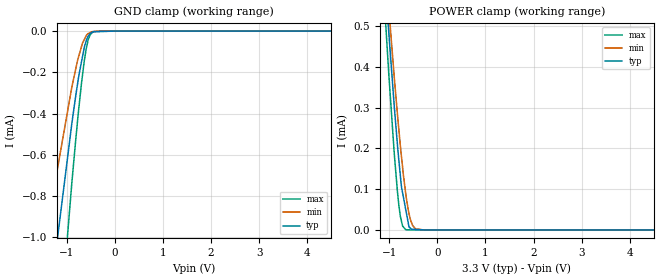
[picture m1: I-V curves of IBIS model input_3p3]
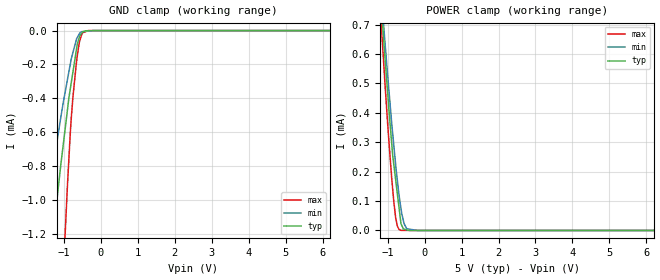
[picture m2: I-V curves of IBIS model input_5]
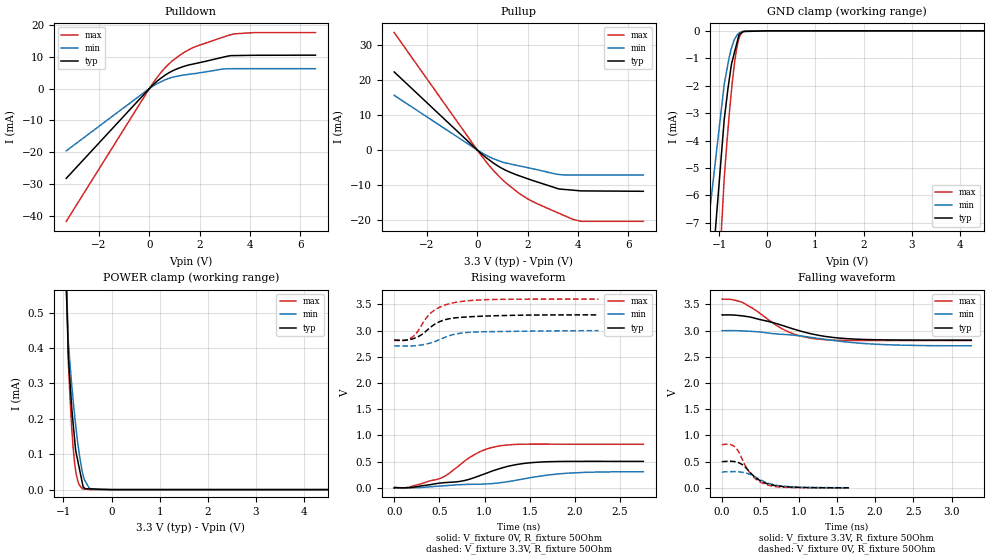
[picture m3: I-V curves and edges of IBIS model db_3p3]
|Texas Instruments Incorporated
| 16-Bit, 2MSPS ADC with P8/P16 Parallel Output, Internal Clock & Internal
| Reference
| Marketing part#   Digital Voltage Range   Package-type   #pins
| ADS8411IBPFBR   2.7V - 5.25V   TQFP   48
| ADS8411IBPFBRG4   2.7V - 5.25V   TQFP   48
| ADS8411IBPFBT   2.7V - 5.25V   TQFP   48
| ADS8411IBPFBTG4   2.7V - 5.25V   TQFP   48
| ADS8411IPFBT   2.7V - 5.25V   TQFP   48
| ADS8411IPFBTG4   2.7V - 5.25V   TQFP   48
[IBIS Ver]   3.2
[File name]   ads8411.ibs
|SIMDE Ver   V3.0 - 201101 - RHL4 - Build 457
[File Rev]   1.0
[Date]   7/21/2011
[Source]
| Texas Instruments Incorporated.
| Analog-eLab Design Center, HPA
| 12500 TI Blvd
| Dallas, TX -75243
| e-mail: elab_scm_ibis@list.ti.com
[Notes]   Revision History:
| Rev 1.0: 7/21/2011
| - Initial version of the model
| - Model generated from simulations in TISPICE
| - Model matched to SPICE simulation
| - C_comp although listed in numerical order of value are
|   obtained from varying PVT conditions. For PVT conditions for
|   each specific value refer the buffer description under
|   respective [Model]. IBIS model user is responsible for using
|   appropriate C_comp to simulate for Signal Integrity.
| - Model names with a trailing _3p3 contains the model for
|   3.3V [3.0V and 3.6V]. Model names with a trailing _5 contains
|   the model for 5.0V [4.5V and 5.5V].
| - Relative part of ADS8412.
|*   EXCEPTION:   *
|*   - Because of the resistor network connected to pad,there will  *
|*   be a leakage current in the Pullup table MAX corner of busy_5*
|*   & POWER CLAMP IV table MAX corners db_5 and db4to11_5 models.*
[Disclaimer]
| This model is designed as an aid for customers of Texas Instruments.
| TI and its licensors and suppliers make no warranties, either expressed
| or implied, with respect to this  model, including the warranties of
| merchantability or fitness for a particular purpose. The model is
| provided solely on an "as is" basis. The entire risk as to its quality
| and performance is with the customer.
[Copyright]
 (C) Copyright 2011 Texas Instruments Incorporated.All rights reserved.
|   ADS8411
[Component]   ADS8411
[Manufacturer]   TI
[Package]   |48 TQFP   -  PFB package
|   typ   min   max
R_pkg   0.07474   0.04062   0.08595
L_pkg   2.62799nH   2.23868nH   3.44226nH
C_pkg   0.45808pF   0.38230pF   0.56945pF
[Pin]  signal_name   model_name   R_pin   L_pin   C_pin
1   REFIN   TERM   0.08206   3.37721nH  0.55796pF
2   REFOUT   TERM   0.07311   2.63474nH  0.48712pF
3   NC   NC   0.06827   2.49388nH  0.46543pF
4   VA+   POWER   0.06574   2.45218nH  0.45840pF
5   AGND   GND   0.06538   2.26018nH  0.41356pF
6   IN+   TERM   0.06584   2.24077nH  0.38230pF
7   IN-   TERM   0.06683   2.25918nH  0.38313pF
8   AGND   GND   0.06727   2.29722nH  0.41664pF
9   VA+   POWER   0.07011   2.54080nH  0.46468pF
10   VA+   POWER   0.07450   2.61853nH  0.47441pF
11   AGND   GND   0.08090   2.78937nH  0.50097pF
12   AGND   GND   0.02781   2.88082nH  0.62037pF
13   VA+   POWER   0.08724   3.49123nH  0.55959pF
14   AGND   GND   0.08150   2.80909nH  0.48998pF
15   AGND   GND   0.08471   2.82596nH  0.47804pF
16   DB15   DB   0.08265   2.78879nH  0.47897pF
17   DB14   DB   0.08081   2.56943nH  0.43166pF
18   DB13   DB   0.08007   2.52568nH  0.39763pF
19   DB12   DB   0.07920   2.50619nH  0.39700pF
20   DB11   DB4to11   0.07811   2.51437nH  0.42861pF
21   DB10   DB4to11   0.07805   2.69832nH  0.47285pF
22   DB9   DB4to11   0.07892   2.71042nH  0.47434pF
23   DB8   DB4to11   0.08131   2.80113nH  0.49547pF
24   VBD+   POWER   0.08699   3.47547nH  0.56533pF
25   BDGND   GND   0.09181   3.57831nH  0.56951pF
26   DB7   DB4to11   0.08145   2.80544nH  0.49887pF
27   DB6   DB4to11   0.07496   2.62998nH  0.47483pF
28   DB5   DB4to11   0.07046   2.54788nH  0.46573pF
29   DB4   DB4to11   0.06751   2.30378nH  0.41738pF
30   DB3   DB   0.06637   2.25187nH  0.38313pF
31   DB2   DB   0.06583   2.23868nH  0.38275pF
32   DB1   DB   0.06587   2.26752nH  0.41559pF
33   DB0   DB   0.06778   2.49130nH  0.46143pF
34   VBD+   POWER   0.07134   2.55123nH  0.46971pF
35   BDGND   GND   0.07672   2.70037nH  0.49534pF
36   BUSY   BUSY   0.08595   3.44226nH  0.56945pF
37   VBD+   POWER   0.08902   3.51744nH  0.56277pF
38   _RESET   INPUT   0.08223   2.81495nH  0.49515pF
39   BYTE   INPUT   0.07913   2.70647nH  0.47619pF
40   _CONVST   INPUT   0.07793   2.68782nH  0.47314pF
41   _RD   INPUT   0.07804   2.50508nH  0.42870pF
42   _CS   INPUT   0.07951   2.50501nH  0.39774pF
43   VA+   POWER   0.08105   2.53403nH  0.39929pF
44   AGND   GND   0.08220   2.58618nH  0.42997pF
45   AGND   GND   0.07817   2.69201nH  0.46931pF
46   VA+   POWER   0.07884   2.69863nH  0.47572pF
47   REFM   TERM   0.04062   2.38885nH  0.53583pF
48   REFM   TERM   0.08222   3.37069nH  0.56325pF
|   Model Selectors
[Model Selector] INPUT
input_3p3  3.3V digital input
input_5   5.0V digital input
[Model Selector] BUSY
busy_3p3   3.3V digital output
busy_5   5.0V digital output
[Model Selector] DB
db_3p3   3.3V 3-state output
db_5   5.0V 3-state output
[Model Selector] DB4to11
db4to11_3p3   3.3V 3-state output
db4to11_5   5.0V 3-state output
[Model Selector] TERM
term_3-3V  3.3V nominal termination
term_5-0V  5.0V nominal termination
[Model] term_3-3V
Model_type Terminator
C_comp   1.0e-20F  1.0e-20F  1.0e-20F
|   typ   min   max
[Voltage Range]   3.3V   3.0V   3.6V
[POWER Clamp Reference]   3.3V   3.0V   3.6V
[GND Clamp Reference]   0V   0V   0V
|Ambient Temperature   25   85   -40
|Junction Temperature
[Temperature Range]   40   100   -40
[Model] term_5-0V
Model_type Terminator
C_comp   1.0e-20F  1.0e-20F  1.0e-20F
|   typ   min   max
[Voltage Range]   5.0V   4.75V   5.25V
[POWER Clamp Reference]   5.0V   4.75V   5.25V
[GND Clamp Reference]   0V   0V   0V
|Ambient Temperature   25   85   -40
|Junction Temperature
[Temperature Range]   40   100   -40
| Models and submodels in the file (10): input_3p3 (Input), input_5 (Input), db_3p3 (3-state), db_5 (3-state), db4to11_3p3 (3-state), db4to11_5 (3-state), busy_3p3 (Output), busy_5 (Output), term_3-3V (Terminator), term_5-0V (Terminator)
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|   input_3p3 Model
[Model]   input_3p3
Model_type   Input
Vinl = 0.8
Vinh = 2.3
|   typ   min   max
|   (nom PVT)   (fast PVT)   (slow PVT)
|C_comp from frequency sweep method (F=1MHz)
|Average
|C_comp   2.437e-12   2.379e-12   2.445e-12
|C_comp from LC tank measurement(L=1nH)
|Average
|Resonant Frequency(Hz)   3.580e+09   3.600e+09   3.550e+09
C_comp   1.978e-12   1.956e-12   2.012e-12
| Where nom  PVT is Nominal Process, 3.3V, 40C
|   Fast PVT is Strong Process,  3.6V, -40C
|   Slow PVT is Weak Process,   3V, 100C
[Model Spec]
Vinh   2.3   2.0   2.6
[Voltage Range]   3.3   3   3.6
|Ambient Temperature   25   85   -40
|Junction Temperature
[Temperature Range]   40   100   -40
[Power Clamp Reference]   3.3   3   3.6
[GND Clamp Reference]   0   0   0
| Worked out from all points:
|   GND clamp passes 1 mA (typ) near -1.19 V on its own axis
|   POWER clamp passes 1 mA (typ) near -1.31 V on its own axis
[GND Clamp]
|   Voltage   I(typ)   I(min)   I(max)
-3.3V     -5.989mA   -4.026mA   -11.09mA
-1.561V   -1.759mA   -1.203mA   -2.732mA
-1.26V    -1.141mA   -754.9uA   -1.788mA
-1.191V   -999.8uA   -663.8uA   -1.581mA
-897.6mV  -451.9uA   -274.2uA   -742.2uA
-752.4mV  -219.8uA   -122.3uA   -378.7uA
-691.2mV  -145.1uA   -72.4uA    -245.9uA
-640.8mV  -84.92uA   -42.96uA   -151.8uA
-597.6mV  -48.27uA   -23.13uA   -86.98uA
-558mV    -25.78uA   -12.14uA   -44.62uA
-471mV    -5.465uA   -2.721uA   -6.698uA
6.6V      0A         0A         0A
[POWER Clamp]
|   Voltage   I(typ)   I(min)   I(max)
-3.3V     4.863mA    4.572mA    5.323mA
-1.159V   738uA      777.9uA    667uA
-1.035V   523.5uA    580.1uA    428.9uA
-1.012V   486uA      545.3uA    384uA
-896.4mV  302.7uA    373.8uA    186.6uA
-802.8mV  172.8uA    247.7uA    62.16uA
-745.8mV  104.9uA    178.4uA    20.9uA
-658.8mV  50.38uA    89.49uA    921.5nA
-590.7mV  7.702uA    39.87uA    227.2nA
-513mV    1.843uA    10.64uA    0A
-285mV    155.8nA    42.15nA    0A
6.6V      0A         0A         0A
|   input_5 Model
[Model]   input_5
Model_type   Input
Vinl = 0.8
Vinh = 4.0
|   typ   min   max
|   (nom PVT)   (fast PVT)   (slow PVT)
|C_comp from frequency sweep method (F=1MHz)
|Average
|C_comp   2.380e-12   2.336e-12   2.422e-12
|C_comp from LC tank measurement(L=1nH)
|Average
|Resonant Frequency(Hz)   3.580e+09   3.600e+09   3.550e+09
C_comp   1.978e-12   1.956e-12   2.012e-12
| Where nom  PVT is Nominal Process, 5V, 40C
|   Fast PVT is Strong Process,  5.25V, -40C
|   Slow PVT is Weak Process,   4.75V, 100C
[Model Spec]
Vinh   4.0   3.75   4.25
[Voltage Range]   5   4.75   5.25
|Ambient Temperature   25   85   -40
|Junction Temperature
[Temperature Range]   40   100   -40
[Power Clamp Reference]   5   4.75   5.25
[GND Clamp Reference]   0   0   0
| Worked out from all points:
|   GND clamp passes 1 mA (typ) near -1.19 V on its own axis
|   POWER clamp passes 1 mA (typ) near -1.31 V on its own axis
[GND Clamp]
|   Voltage   I(typ)   I(min)   I(max)
-5V       -11.75mA   -8.078mA   -27.34mA
-1.717V   -2.121mA   -1.453mA   -5.102mA
-1.306V   -1.23mA    -821uA     -2.898mA
-1.003V   -645.1uA   -405.9uA   -1.365mA
-903mV    -465uA     -287.6uA   -907.2uA
-824.3mV  -339.6uA   -194.1uA   -593.4uA
-756mV    -244.3uA   -129.5uA   -391.6uA
-640.5mV  -83uA      -41.72uA   -151.3uA
-582.7mV  -40.19uA   -19.54uA   -69.03uA
-517.8mV  -14.97uA   -6.289uA   -21.97uA
-341.2mV  -868.4nA   -2.903uA   -50.26nA
10V       0A         0A         0A
[POWER Clamp]
|   Voltage   I(typ)   I(min)   I(max)
-5V       8.258mA    7.712mA    9.133mA
-1.306V   999.6uA    1.019mA    965uA
-1.088V   612.7uA    662.6uA    529uA
-971.2mV  419.3uA    483.8uA    311.5uA
-865mV    256.6uA    330.8uA    141.3uA
-834.7mV  225.2uA    290.8uA    98.93uA
-740.2mV  127.1uA    173.1uA    15.74uA
-640.5mV  23.57uA    75.6uA     443.5nA
-555.7mV  4.548uA    23.31uA    384.9nA
-484.5mV  2.269uA    5.873uA    335.5nA
-190mV    0A         0A         131.6nA
10V       0A         0A         0A
|   db_3p3 Model
[Model]   db_3p3
Model_type   3-state
Polarity   Non-Inverting
Vmeas = 1.65
Vref = 1.65
Cref = 20pF
Rref = 50
|   typ   min   max
|   (nom PVT)   (fast PVT)   (slow PVT)
|C_comp from frequency sweep method (F=1MHz)
|C_comp   3.371e-12   3.312e-12   3.431e-12
|ON state : BUFFER OUTPUT TURNED HIGH
|C_comp   3.371e-12   3.312e-12   3.431e-12
|OFF state: BUFFER IN HIGH IMPEDANCE
|C_comp   3.336e-12   3.283e-12   3.394e-12
|C_comp from LC tank measurement(L=1nH)
|Resonant Frequency(Hz)   3.050e+09   3.070e+09   3.000e+09
C_comp   2.726e-12   2.690e-12   2.817e-12
|ON state : BUFFER OUTPUT TURNED HIGH
|Resonant Frequency(Hz)   3.050e+09   3.070e+09   3.010e+09
|C_comp   2.726e-12   2.690e-12   2.799e-12
|OFF state: BUFFER IN HIGH IMPEDANCE
|Resonant Frequency(Hz)   3.050e+09   3.070e+09   3.000e+09
|C_comp   2.726e-12   2.690e-12   2.817e-12
| Where nom  PVT is Nominal Process, 3.3V, 40C
|   Fast PVT is Strong Process,  3.6V, -40C
|   Slow PVT is Weak Process,   3V, 100C
[Voltage Range]   3.3   3   3.6
|Ambient Temperature   25   85   -40
|Junction Temperature
[Temperature Range]   40   100   -40
[Pullup Reference]   3.3   3   3.6
[Pulldown Reference]   0   0   0
[Power Clamp Reference]   3.3   3   3.6
[GND Clamp Reference]   0   0   0
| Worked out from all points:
|   slope of the pulldown table from 0 to 0.495 V, typ, clamps not added: 143 ohm
|   slope of the pullup table from 0 to 0.495 V, typ, clamps not added: 168 ohm
|   GND clamp passes 1 mA (typ) near -0.72 V on its own axis
|   falling waveform, V_fixture 3.3V, R_fixture 50Ohm: 20-80 % time 731ps typ, 1.07ns min, 501ps max; typ from 3.3 V to 2.82 V
|   rising waveform, V_fixture 0V, R_fixture 50Ohm: 20-80 % time 674ps typ, 972ps min, 439ps max; typ from 0 V to 0.505 V
|   rising waveform, V_fixture 3.3V, R_fixture 50Ohm: 20-80 % time 261ps typ, 298ps min, 244ps max; typ from 2.82 V to 3.3 V
|   falling waveform, V_fixture 0V, R_fixture 50Ohm: 20-80 % time 252ps typ, 284ps min, 219ps max; typ from 0.505 V to 0.001 V
[Pulldown]
|   Voltage   I(typ)   I(min)   I(max)
-3.3V     -28.14mA   -19.51mA   -41.61mA
126mV     1.005mA    697.4uA    1.535mA
478.8mV   3.358mA    2.196mA    5.234mA
939.6mV   5.626mA    3.599mA    8.872mA
1.372V    6.953mA    4.268mA    11.31mA
1.706V    7.639mA    4.605mA    12.76mA
2.934V    9.846mA    6.13mA     16.14mA
3.344V    10.34mA    6.23mA     17.13mA
4.162V    10.44mA    6.251mA    17.56mA
6.6V      10.48mA    6.251mA    17.56mA
[GND Clamp]
|   Voltage   I(typ)   I(min)   I(max)
-3.3V     -645.3mA   -463.1mA   -985.5mA
-1.541V   -17.34mA   -11.8mA    -25.88mA
-897.6mV  -3.244mA   -1.959mA   -5.39mA
-835.2mV  -2.336mA   -1.359mA   -3.937mA
-745.8mV  -1.209mA   -630.6uA   -2.167mA
-730.8mV  -1.107mA   -544.2uA   -1.895mA
-684mV    -787uA     -310.8uA   -1.181mA
-640.8mV  -491.9uA   -186uA     -668.9uA
-590.7mV  -149.7uA   -84.2uA    -285.4uA
-558mV    -100.6uA   -50.98uA   -133.5uA
-360mV    -18.27uA   -912.9nA   -156.2nA
6.6V      0A         0A         0A
[Pullup]
|   Voltage   I(typ)   I(min)   I(max)
-3.3V     22.37mA    15.66mA    33.65mA
172.8mV   -1.117mA   -764.9uA   -1.711mA
543.6mV   -3.215mA   -2.181mA   -5.053mA
939.6mV   -5.084mA   -3.294mA   -8.094mA
1.649V    -7.339mA   -4.529mA   -12.33mA
2.167V    -8.656mA   -5.311mA   -14.62mA
3.241V    -11.16mA   -7.006mA   -18.11mA
3.809V    -11.52mA   -7.192mA   -19.9mA
4.133V    -11.72mA   -7.192mA   -20.43mA
6.6V      -11.83mA   -7.192mA   -20.43mA
[POWER Clamp]
|   Voltage   I(typ)   I(min)   I(max)
-3.3V     638.7mA    457.7mA    976.4mA
-1.523V   3.32mA     2.55mA     4.556mA
-897.6mV  375.3uA    417.9uA    364.2uA
-864mV    305.6uA    355.7uA    261uA
-831.6mV  238.4uA    301.9uA    181.9uA
-770.4mV  146.2uA    214.1uA    78.28uA
-745.8mV  110.5uA    182.3uA    53.42uA
-702mV    81.49uA    131.6uA    24.44uA
-601.2mV  14.79uA    46.65uA    2.01uA
-459mV    2.105uA    3.326uA    248.6nA
-285mV    1.301uA    42.46nA    0A
6.6V      0A         0A         0A
[Ramp]
R_load = 50
|   typ   min   max
dV/dt_r   0.303298/6.73839e-10   0.184837/9.72111e-10   0.498804/4.3692e-10
dV/dt_f   0.289442/7.30259e-10   0.175777/1.07562e-09   0.474129/5.0075e-10
[Falling Waveform]
V_fixture = 3.3V
V_fixture_min = 3V
V_fixture_max = 3.6V
R_fixture = 50Ohm
|   Time   V(typ)   V(min)   V(max)
0s        3.3V       3V         3.6V
134ps     3.298V     3V         3.589V
268ps     3.28V      2.994V     3.535V
807ps     3.089V     2.927V     3.017V
989ps     3.006V     2.904V     2.91V
1.172ns   2.936V     2.869V     2.852V
1.456ns   2.868V     2.811V     2.818V
1.815ns   2.833V     2.758V     2.81V
2.276ns   2.82V      2.724V     2.81V
3.258ns   2.818V     2.709V     2.81V
[Rising Waveform]
V_fixture = 0V
V_fixture_min = 0V
V_fixture_max = 0V
R_fixture = 50Ohm
|   Time   V(typ)   V(min)   V(max)
0s        1.364nV    2.286nV    1.294nV
157ps     3.568mV    799uV      10.49mV
516ps     92.61mV    35.37mV    184.8mV
739ps     126.4mV    61.6mV     454.1mV
883ps     192.4mV    68.51mV    629.2mV
1.162ns   363.7mV    95.39mV    798.9mV
1.378ns   451.4mV    154mV      830.7mV
1.653ns   495.6mV    233.1mV    834.2mV
2.108ns   505.6mV    295.7mV    831.6mV
2.759ns   505.4mV    307.5mV    831.3mV
[Rising Waveform]
V_fixture = 3.3V
V_fixture_min = 3V
V_fixture_max = 3.6V
R_fixture = 50Ohm
|   Time   V(typ)   V(min)   V(max)
0s        2.818V     2.707V     2.81V
105ps     2.815V     2.705V     2.81V
185ps     2.833V     2.706V     2.858V
248ps     2.871V     2.713V     2.954V
340ps     2.971V     2.738V     3.203V
411ps     3.075V     2.769V     3.343V
532ps     3.19V      2.85V      3.467V
647ps     3.236V     2.921V     3.527V
1.014ns   3.277V     2.979V     3.59V
2.263ns   3.3V       2.999V     3.6V
[Falling Waveform]
V_fixture = 0V
V_fixture_min = 0V
V_fixture_max = 0V
R_fixture = 50Ohm
|   Time   V(typ)   V(min)   V(max)
0s        505.5mV    308.1mV    831.3mV
105ps     507.6mV    309.6mV    828.1mV
176ps     497.4mV    309.6mV    769.5mV
219ps     478.1mV    305.9mV    682.1mV
270ps     436.1mV    296mV      523.6mV
366ps     295.6mV    256.5mV    282.8mV
456ps     175.3mV    190.5mV    151.8mV
561ps     94.17mV    111.7mV    70.91mV
889ps     15.93mV    21.5mV     5.59mV
1.657ns   822.3uV    2.265mV    33.05uV
